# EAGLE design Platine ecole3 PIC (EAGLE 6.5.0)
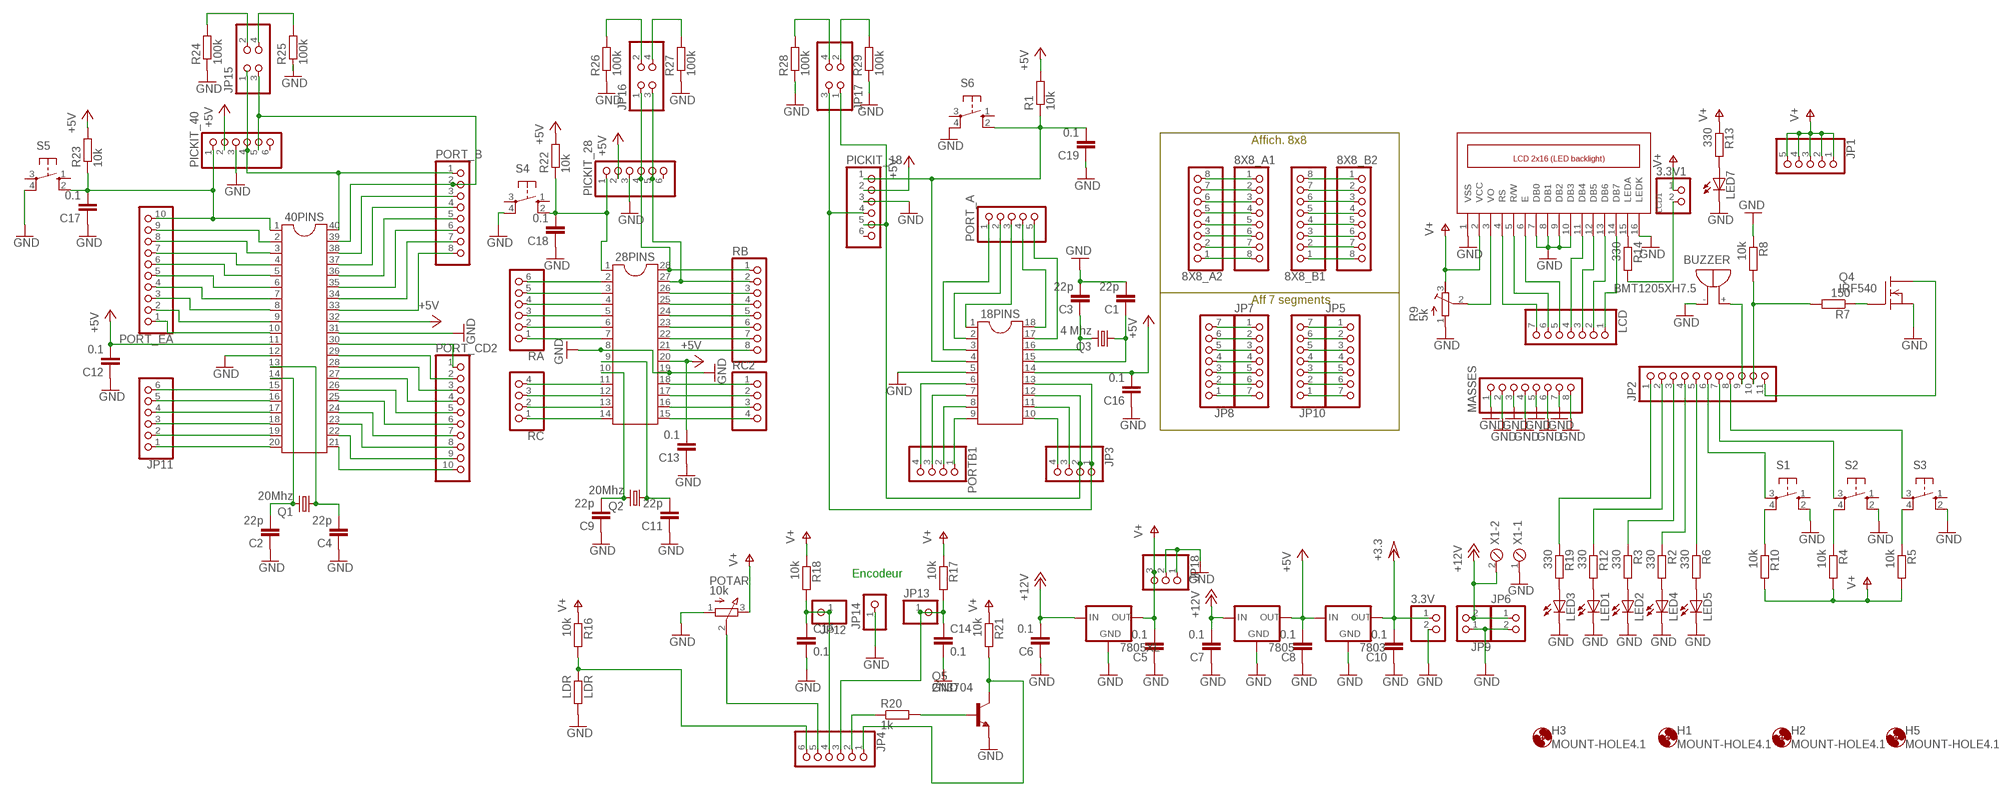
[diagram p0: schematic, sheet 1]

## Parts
3.3V  PINHD-1X2  [1X02]
3.3V1  PINHD-1X2  [1X02]
8X8_A1  PINHD-1X8/LONG  [1X08]
8X8_A2  PINHD-1X8/LONG  [1X08]
8X8_B1  PINHD-1X8/LONG  [1X08]
8X8_B2  PINHD-1X8/LONG  [1X08]
18PINS  DIL18  [DIL18]
28PINS  DIL28-3  [DIL28-3]
40PINS  DIL40  [DIL40]
7803  78LXX  [78LXX]
7805  78LXX  [78LXX]
7805XL  78XXL  [78XXL]
BUZZER  BMT1205XH7.5  [BMT1205XH7.5]
C1  22p  C-EU050-025X075  [C050-025X075]
C2  22p  C-EU050-025X075  [C050-025X075]
C3  22p  C-EU050-025X075  [C050-025X075]
C4  22p  C-EU050-025X075  [C050-025X075]
C5  0.1  C-EU050-025X075  [C050-025X075]
C6  0.1  C-EU050-025X075  [C050-025X075]
C7  0.1  C-EU050-025X075  [C050-025X075]
C8  0.1  C-EU050-025X075  [C050-025X075]
C9  22p  C-EU050-025X075  [C050-025X075]
C10  0.1  C-EU050-025X075  [C050-025X075]
C11  22p  C-EU050-025X075  [C050-025X075]
C12  0.1  C-EU050-025X075  [C050-025X075]
C13  0.1  C-EU050-025X075  [C050-025X075]
C14  0.1  C-EU075-032X103  [C075-032X103]
C15  0.1  C-EU075-032X103  [C075-032X103]
C16  0.1  C-EU050-025X075  [C050-025X075]
C17  0.1  C-EU050-025X075  [C050-025X075]
C18  0.1  C-EU050-025X075  [C050-025X075]
C19  0.1  C-EU050-025X075  [C050-025X075]
H1  MOUNT-HOLE4.1  [4,1]
H2  MOUNT-HOLE4.1  [4,1]
H3  MOUNT-HOLE4.1  [4,1]
H5  MOUNT-HOLE4.1  [4,1]
JP1  PINHD-1X5  [1X05]
JP2  PINHD-1X11  [1X11]
JP3  PINHD-1X4  [1X04]
JP4  PINHD-1X6  [1X06]
JP5  PINHD-1X7  [1X07]
JP6  PINHD-1X2  [1X02]
JP7  PINHD-1X7  [1X07]
JP8  PINHD-1X7  [1X07]
JP9  PINHD-1X2  [1X02]
JP10  PINHD-1X7  [1X07]
JP11  PINHD-1X6  [1X06]
JP12  PINHD-1X1  [1X01]
JP13  PINHD-1X1  [1X01]
JP14  PINHD-1X1  [1X01]
JP15  PINHD-2X2  [2X02]
JP16  PINHD-2X2  [2X02]
JP17  PINHD-2X2  [2X02]
JP18  PINHD-1X3  [1X03]
LCD  PINHD-1X7/LONG  [1X07]
LCD1  LCD_2X16_SIL  [HY-1602F]
LDR  LDR  R-EU_0207/7  [0207/7]
LED1  LED5MM  [LED5MM]
LED2  LED5MM  [LED5MM]
LED3  LED5MM  [LED5MM]
LED4  LED5MM  [LED5MM]
LED5  LED5MM  [LED5MM]
LED7  LED3MM  [LED3MM]
MASSES  PINHD-1X8/LONG  [1X08]
PICKIT_18  PINHD-1X6  [1X06]
PICKIT_28  PINHD-1X6  [1X06]
PICKIT_40  PINHD-1X6  [1X06]
PORT_A  PINHD-1X5  [1X05]
PORT_B  PINHD-1X8  [1X08]
PORT_CD2  PINHD-1X10  [1X10]
PORT_EA  PINHD-1X10  [1X10]
PORTB1  PINHD-1X4  [1X04]
POTAR  10k  EVUF2A  [EVUF]
Q1  20Mhz  CRYSTALHC49S  [HC49/S]
Q2  20Mhz  CRYSTALHC49S  [HC49/S]
Q3  4 Mhz  CRYSTALHC49S  [HC49/S]
Q4  IRF540  [TO220]
Q5  2N3704  [TO92]
R1  10k  R-EU_0207/7  [0207/7]
R2  330  R-EU_0207/7  [0207/7]
R3  330  R-EU_0207/7  [0207/7]
R4  10k  R-EU_0207/7  [0207/7]
R5  10k  R-EU_0207/7  [0207/7]
R6  330  R-EU_0207/7  [0207/7]
R7  150  R-EU_0207/7  [0207/7]
R8  10k  R-EU_0207/7  [0207/7]
R9  5k  R-TRIMM3339P  [RTRIM3339P]
R10  10k  R-EU_0207/7  [0207/7]
R12  330  R-EU_0207/7  [0207/7]
R13  330  R-EU_0207/7  [0207/7]
R14  330  R-EU_0207/7  [0207/7]
R16  10k  R-EU_0207/7  [0207/7]
R17  10k  R-EU_0207/7  [0207/7]
R18  10k  R-EU_0207/7  [0207/7]
R19  330  R-EU_0207/7  [0207/7]
R20  1k  R-EU_0207/7  [0207/7]
R21  10k  R-EU_0207/7  [0207/7]
R22  10k  R-EU_0207/7  [0207/7]
R23  10k  R-EU_0207/7  [0207/7]
R24  100k  R-EU_0207/7  [0207/7]
R25  100k  R-EU_0207/7  [0207/7]
R26  100k  R-EU_0207/7  [0207/7]
R27  100k  R-EU_0207/7  [0207/7]
R28  100k  R-EU_0207/7  [0207/7]
R29  100k  R-EU_0207/7  [0207/7]
RA  PINHD-1X6  [1X06]
RB  PINHD-1X8  [1X08]
RC  PINHD-1X4  [1X04]
RC2  PINHD-1X4  [1X04]
S1  10-XX  [B3F-10XX]
S2  10-XX  [B3F-10XX]
S3  10-XX  [B3F-10XX]
S4  10-XX  [B3F-10XX]
S5  10-XX  [B3F-10XX]
S6  10-XX  [B3F-10XX]
X1  MPT2  [2POL254]

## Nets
8X8_A1: 8X8_A1.1 8X8_A2.8
+5V: 18PINS.14 28PINS.20 40PINS.11 40PINS.32 7803.IN 7805.OUT C8.2 C12.2 C13.2 C16.2 PICKIT_18.2 PICKIT_28.2 PICKIT_40.2 R1.2 R22.2 R23.2
+12V: 7805.IN 7805XL.IN C6.2 C7.2 JP6.1 JP9.2 X1.2
GND: 3.3V.2 18PINS.5 28PINS.8 28PINS.19 40PINS.12 40PINS.31 7803.GND 7805.GND 7805XL.GND BUZZER.- C1.2 C2.1 C3.2 C4.1 C5.1 C6.1 C7.1 C8.1 C9.1 C10.1 C11.1 C12.1 C13.1 C14.2 C15.2 C16.1 C17.1 C18.1 C19.1 JP6.2 JP9.1 JP14.1 JP18.1 JP18.2 LCD1.1(VSS) LCD1.7(DB0) LCD1.8(DB1) LCD1.9(DB2) LCD1.10(DB3) LCD1.16(LEDK) LDR.2 LED1.K(C) LED2.K(C) LED3.K(C) LED4.K(C) LED5.K(C) LED7.K(C) MASSES.1 MASSES.2 MASSES.3 MASSES.4 MASSES.5 MASSES.6 MASSES.7 MASSES.8 PICKIT_18.3 PICKIT_28.3 PICKIT_40.3 POTAR.1(A) Q4.3(S) Q5.3(E) R8.1 R9.1(A) R24.1 R25.1 R26.1 R27.1 R28.1 R29.1 S1.2(S1) S2.2(S1) S3.2(S1) S4.4(P1) S5.4(P1) S6.4(P1) X1.1
LED_POUSS: JP2.2 R12.1
N$1: 18PINS.16 C3.1 Q3.2
N$2: 18PINS.11 JP3.3
N$3: 18PINS.15 C1.1 Q3.1
N$4: 18PINS.10 JP3.4
N$5: 18PINS.13 JP3.1 JP17.3 PICKIT_18.4
N$7: 18PINS.9 PORTB1.1
N$9: 18PINS.7 PORTB1.3
N$10: 18PINS.6 PORTB1.4
N$11: 18PINS.17 PORT_A.5
N$12: 18PINS.18 PORT_A.4
N$13: 18PINS.1 PORT_A.3
N$14: 18PINS.2 PORT_A.2
N$15: 18PINS.3 PORT_A.1
N$16: 40PINS.40 JP15.1 PICKIT_40.4 PORT_B.1
N$17: 18PINS.4 C19.2 PICKIT_18.1 R1.1 S6.2(S1)
N$18: 40PINS.39 JP15.3 PICKIT_40.5 PORT_B.2
N$19: 40PINS.1 C17.2 PICKIT_40.1 PORT_EA.10 R23.1 S5.2(S1)
N$20: LED1.A R12.2
N$21: R4.1 S2.4(P1)
N$22: JP2.11 Q4.2(D)
N$23: R5.1 S3.4(P1)
N$24: LED2.A R3.2
N$25: LED4.A R2.2
N$26: LED5.A R6.2
N$27: R10.1 S1.4(P1)
N$29: JP2.7 S2.3(P)
N$30: JP2.8 S3.3(P)
N$31: JP2.10 R7.2 R8.2
N$32: Q4.1(G) R7.1
N$33: 40PINS.2 PORT_EA.9
N$34: 40PINS.3 PORT_EA.8
N$35: 40PINS.4 PORT_EA.7
N$36: 40PINS.5 PORT_EA.6
N$37: 40PINS.6 PORT_EA.5
N$38: 40PINS.7 PORT_EA.4
N$39: 40PINS.8 PORT_EA.3
N$40: 40PINS.9 PORT_EA.2
N$41: 40PINS.10 PORT_EA.1
N$42: BUZZER.+ JP2.9
N$68: 40PINS.38 PORT_B.3
N$69: 40PINS.37 PORT_B.4
N$70: 40PINS.36 PORT_B.5
N$71: 40PINS.35 PORT_B.6
N$72: 40PINS.34 PORT_B.7
N$73: 40PINS.33 PORT_B.8
N$74: 40PINS.15 JP11.6
N$75: 40PINS.16 JP11.5
N$76: 40PINS.17 JP11.4
N$77: 40PINS.19 JP11.2
N$78: 40PINS.20 JP11.1
N$79: 40PINS.30 PORT_CD2.1
N$80: 40PINS.29 PORT_CD2.2
N$81: 40PINS.27 PORT_CD2.4
N$82: 40PINS.28 PORT_CD2.3
N$83: 40PINS.26 PORT_CD2.5
N$84: 40PINS.25 PORT_CD2.6
N$85: 40PINS.24 PORT_CD2.7
N$86: 40PINS.23 PORT_CD2.8
N$87: 40PINS.22 PORT_CD2.9
N$88: 40PINS.21 PORT_CD2.10
N$89: LCD1.3(VO) R9.2(S)
N$90: 40PINS.14 C2.2 Q1.2
N$91: 40PINS.13 C4.2 Q1.1
N$93: 8X8_A1.2 8X8_A2.7
N$94: 8X8_A1.3 8X8_A2.6
N$95: 8X8_A1.4 8X8_A2.5
N$96: 8X8_A1.5 8X8_A2.4
N$97: 8X8_A1.6 8X8_A2.3
N$98: 8X8_A1.7 8X8_A2.2
N$99: 8X8_A1.8 8X8_A2.1
N$100: 8X8_B1.8 8X8_B2.1
N$101: 8X8_B1.7 8X8_B2.2
N$102: 8X8_B1.6 8X8_B2.3
N$103: 8X8_B1.5 8X8_B2.4
N$104: 8X8_B1.4 8X8_B2.5
N$105: 8X8_B1.3 8X8_B2.6
N$106: 8X8_B1.2 8X8_B2.7
N$107: 8X8_B1.1 8X8_B2.8
N$108: LCD1.11(DB4) LCD.4
N$109: LCD1.4(RS) LCD.7
N$110: LCD1.5(R/W) LCD.6
N$111: LCD1.6(E) LCD.5
N$112: LCD1.12(DB5) LCD.3
N$113: LCD1.13(DB6) LCD.2
N$114: LCD1.14(DB7) LCD.1
N$116: JP2.5 R6.1
N$117: JP2.6 S1.3(P)
N$118: JP2.4 R2.1
N$119: JP2.3 R3.1
N$143: LED7.A R13.2
N$144: LCD1.15(LEDA) R14.1
N$145: 3.3V1.2 R14.2
N$148: JP7.1 JP8.7
N$149: JP7.2 JP8.6
N$150: JP7.3 JP8.5
N$151: JP7.4 JP8.4
N$152: JP7.5 JP8.3
N$153: JP5.1 JP10.7
N$154: JP5.2 JP10.6
N$155: JP5.3 JP10.5
N$156: JP5.4 JP10.4
N$157: JP5.5 JP10.3
N$158: JP7.6 JP8.2
N$159: JP7.7 JP8.1
N$160: JP5.6 JP10.2
N$161: JP5.7 JP10.1
N$166: 28PINS.10 C9.2 Q2.2
N$167: 28PINS.9 C11.2 Q2.1
N$168: 28PINS.2 RA.6
N$170: 28PINS.3 RA.5
N$171: 28PINS.28 JP16.1 PICKIT_28.4 RB.1
N$172: 28PINS.27 JP16.3 PICKIT_28.5 RB.2
N$173: 28PINS.4 RA.4
N$174: 28PINS.5 RA.3
N$175: 28PINS.6 RA.2
N$176: 28PINS.7 RA.1
N$177: 28PINS.11 RC.4
N$178: 28PINS.12 RC.3
N$179: 28PINS.13 RC.2
N$180: 28PINS.14 RC.1
N$181: 28PINS.18 RC2.1
N$182: 28PINS.17 RC2.2
N$183: 28PINS.16 RC2.3
N$184: 28PINS.15 RC2.4
N$185: 28PINS.21 RB.8
N$186: 28PINS.22 RB.7
N$187: 28PINS.23 RB.6
N$188: 28PINS.24 RB.5
N$189: 28PINS.25 RB.4
N$190: 28PINS.26 RB.3
N$196: JP4.5 POTAR.2(S)
N$197: C14.1 JP4.3 JP13.1 R17.2
N$198: C15.1 JP4.4 JP12.1 R18.2
N$199: JP4.6 LDR.1 R16.2
N$206: LED3.A R19.2
N$207: JP2.1 R19.1
N$208: JP4.1 Q5.2(C) R21.2
N$209: Q5.1(B) R20.2
N$210: JP4.2 R20.1
N$211: 40PINS.18 JP11.3
N$213: 28PINS.1 C18.2 PICKIT_28.1 R22.1 S4.2(S1)
N$216: JP15.2 R24.2
N$217: JP15.4 R25.2
N$222: JP16.2 R26.2
N$223: JP16.4 R27.2
N$224: JP17.4 R28.2
N$225: JP17.2 R29.2
PORT_B84: 18PINS.8 PORTB1.2
PORTB2: 18PINS.12 JP3.2 JP17.1 PICKIT_18.5
V+: 3.3V1.1 7805XL.OUT C5.2 JP1.1 JP1.2 JP1.3 JP1.4 JP1.5 JP18.3 LCD1.2(VCC) POTAR.3(E) R4.2 R5.2 R9.3(E) R10.2 R13.1 R16.1 R17.1 R18.1 R21.1
VCC/2: 3.3V.1 7803.OUT C10.2 ; supply symbol labelled +3.3
Unconnected: PICKIT_18.6 PICKIT_28.6 PICKIT_40.6 S1.1(S) S2.1(S) S3.1(S) S4.1(S) S4.3(P) S5.1(S) S5.3(P) S6.1(S) S6.3(P)

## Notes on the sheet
- Affich. 8x8
- Aff 7 segments
- Encodeur

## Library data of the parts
3.3V 3.3V1 JP6 JP9 = pinhead:PINHD-1X2: PIN HEADER
8X8_A1 8X8_A2 8X8_B1 8X8_B2 MASSES = pinhead_v2:PINHD-1X8: PIN HEADER
18PINS = ic-package:DIL18: Dual In Line / Socket
28PINS = ic-package:DIL28: Dual In Line
40PINS = ic-package:DIL40: Dual In Line
7803 7805 = v-reg:78LXX: VOLTAGE REGULATOR
7805XL = v-reg:78XXL: VOLTAGE REGULATOR
BUZZER = buzzer:BMT1205XH7.5: MAGNETIC TRANSDUCER; OC_FARNELL: unknown; OC_NEWARK: unknown
C1-C19 = rcl:C-EU: CAPACITOR, European symbol
H1-H3 H5 = holes:MOUNT-HOLE: MOUNTING HOLE with drill center marker
JP1 PORT_A = pinhead:PINHD-1X5: PIN HEADER
JP2 = pinhead:PINHD-1X11: PIN HEADER
JP3 PORTB1 RC RC2 = pinhead:PINHD-1X4: PIN HEADER
JP4 JP11 PICKIT_18 PICKIT_28 PICKIT_40 RA = pinhead:PINHD-1X6: PIN HEADER
JP5 JP7 JP8 JP10 = pinhead:PINHD-1X7: PIN HEADER
JP12-JP14 = pinhead:PINHD-1X1: PIN HEADER
JP15-JP17 = pinhead:PINHD-2X2: PIN HEADER
JP18 = pinhead:PINHD-1X3: PIN HEADER
LCD = pinhead_v2:PINHD-1X7: PIN HEADER
LCD1 = lcd_2x16_led_backlight:LCD_2X16_SIL
LDR R1-R8 R10 R12-R14 R16-R29 = rcl:R-EU_: RESISTOR, European symbol
LED1-LED5 LED7 = led:LED: LED
PORT_B RB = pinhead:PINHD-1X8: PIN HEADER
PORT_CD2 PORT_EA = pinhead:PINHD-1X10: PIN HEADER
POTAR = pot:EVU: 9 mm Square Rotary Potentiometers Source: Panasonic
Q1-Q3 = crystal:CRYSTAL: CRYSTAL
Q4 = transistor-fet:IRF540: N-Channel Enhancement MOSFET (HEXFET); 100V; 28A; 0,077Ohm
Q5 = transistor-npn:2N3704: NPN Transistor
R9 = rcl:R-TRIMM: Trimm resistor
S1-S6 = switch-omron:10-XX: OMRON SWITCH; MPN: B3F-1000; OC_FARNELL: 176432; OC_NEWARK: 36M3542
X1 = con-phoenix-254:MPT2: PHOENIX CONNECTOR; OC_FARNELL: unknown; OC_NEWARK: unknown

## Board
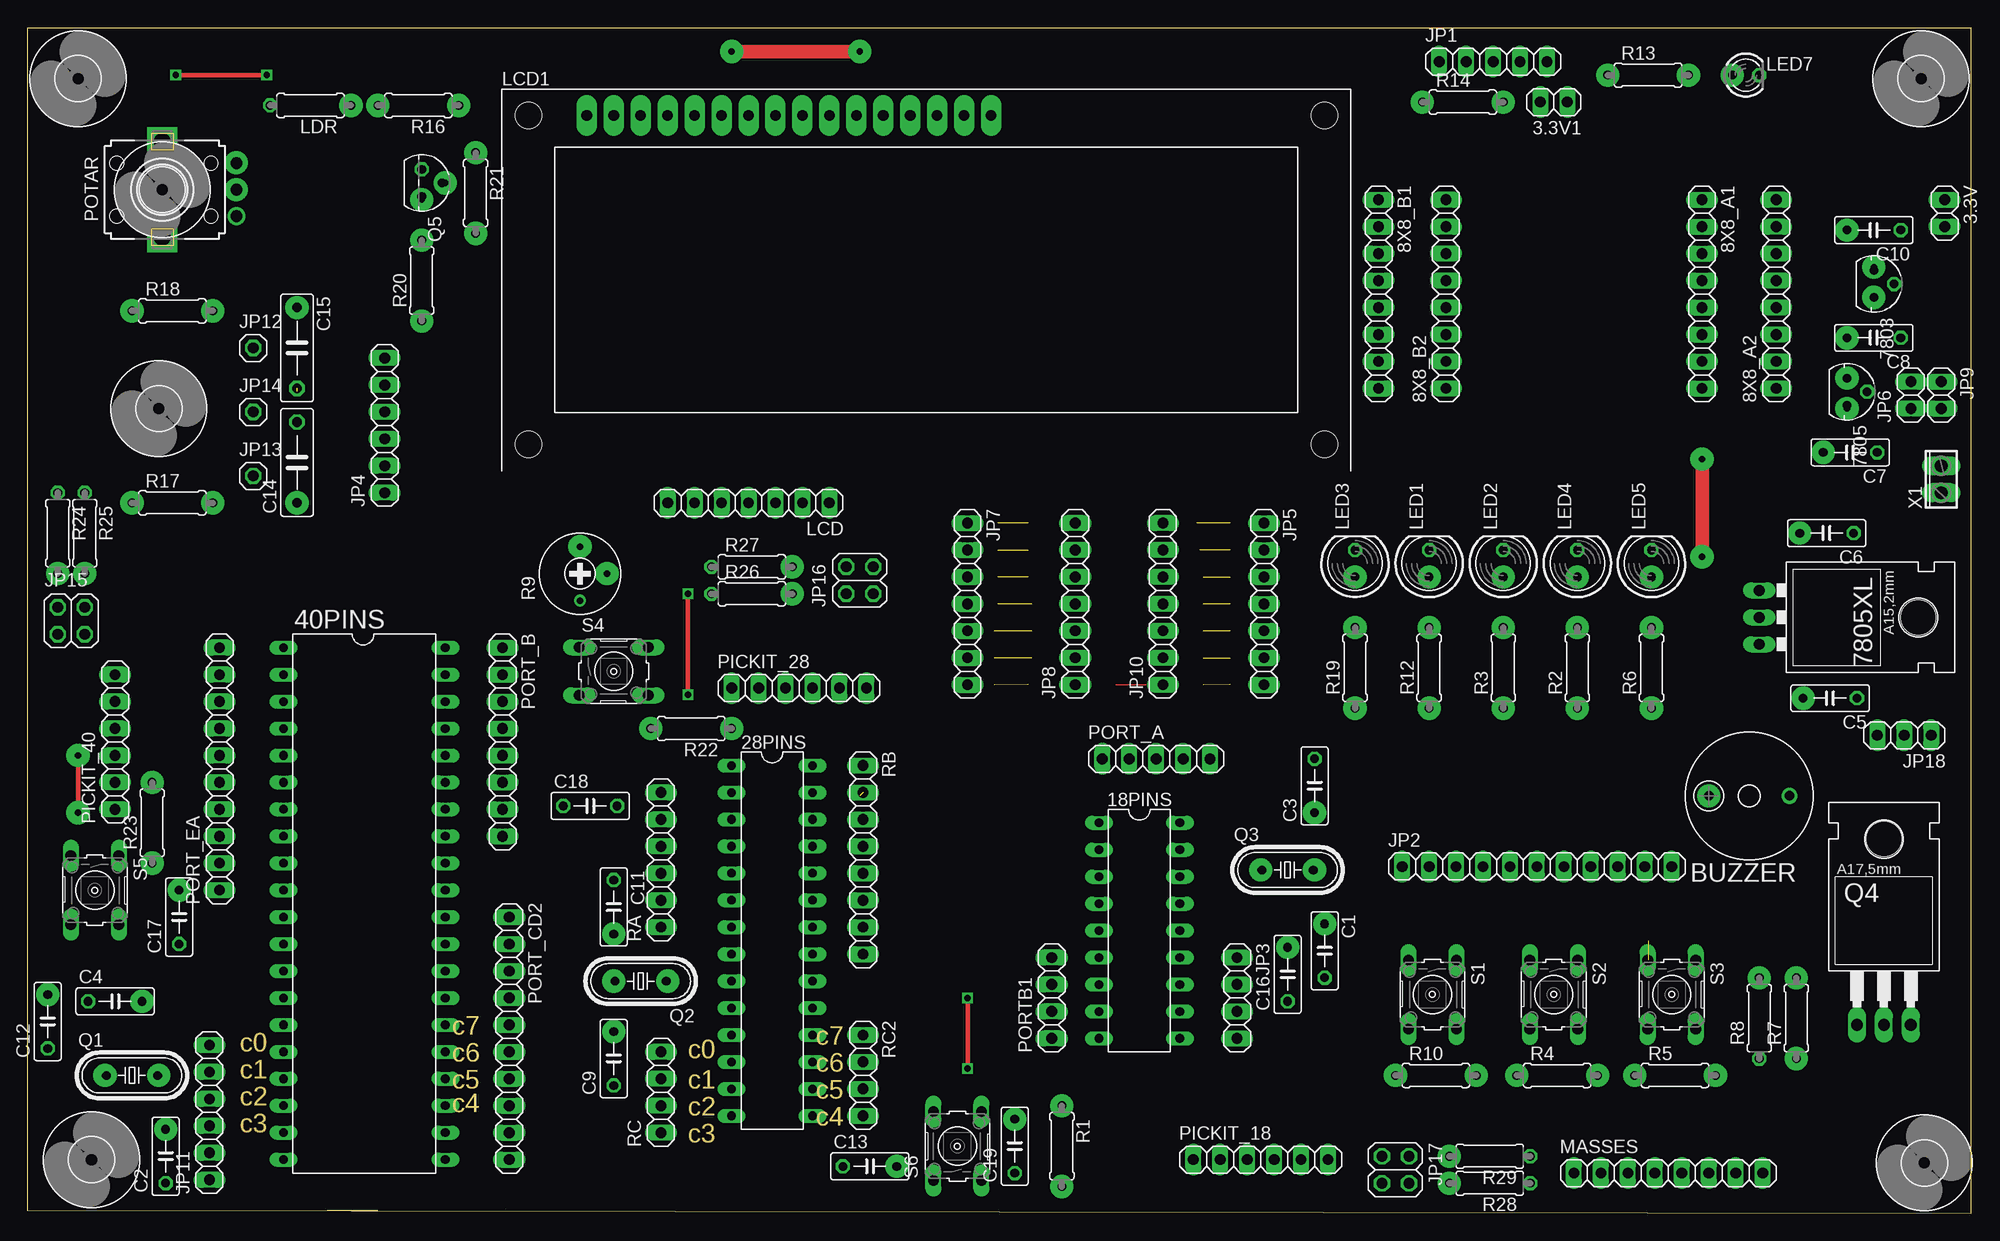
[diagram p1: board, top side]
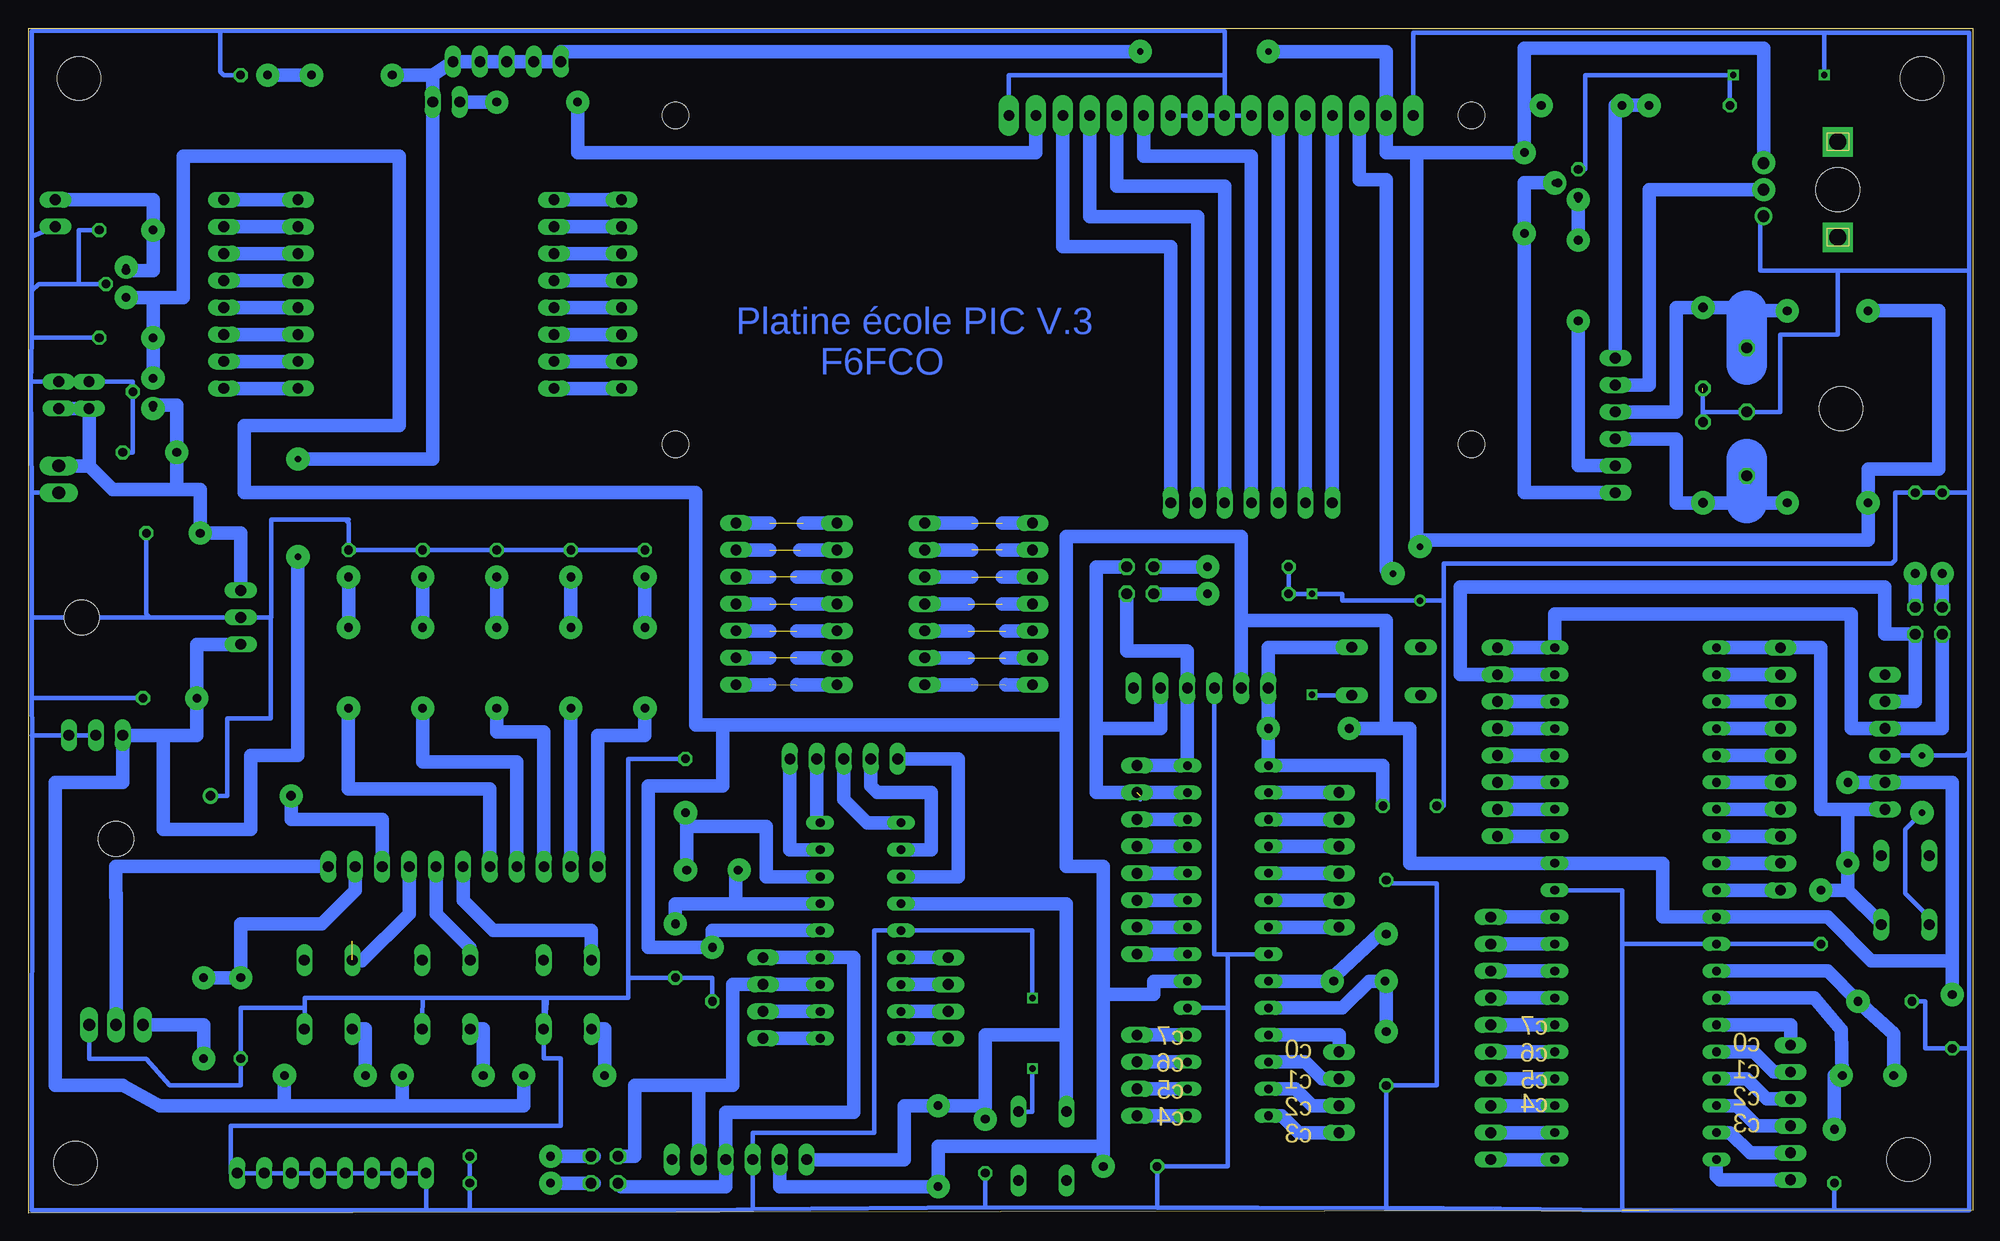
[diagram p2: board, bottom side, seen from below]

Size 183.18 x 111.75 mm. Coordinates in mm from the lower left corner, seen from the top.
Outline: 0,0.32 183.18,0 183.18,111.75 0,111.75 0,0.32
Copper layers (1*16): Top 0.035mm / dielectric 1.5mm / Bottom 0.035mm
Design rules "default": minimum track width 10mil, minimum drill 24mil, track to track 8mil, track to pad 8mil, pad to pad 8mil, via to via 8mil, smd to smd 8mil, copper to edge 40mil, drill to drill 8mil, minimum pad ring 10mil, minimum via ring 8mil, stop-mask expansion 4mil, vias tented up to drill 0mil, thermal gap 10mil

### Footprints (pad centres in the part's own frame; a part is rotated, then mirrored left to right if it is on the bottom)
1X02 = drill 1.016 long: 1 -1.27,0; 2 1.27,0
1X08 = drill 1.016 long: 1 -8.89,0; 2 -6.35,0; 3 -3.81,0; 4 -1.27,0; 5 1.27,0; 6 3.81,0; 7 6.35,0; 8 8.89,0
DIL18 = drill 0.813 long: 1 -10.16,-3.81; 2 -7.62,-3.81; 3 -5.08,-3.81; 4 -2.54,-3.81; 5 0,-3.81; 6 2.54,-3.81; 7 5.08,-3.81; 8 7.62,-3.81; 9 10.16,-3.81; 10 10.16,3.81; 11 7.62,3.81; 12 5.08,3.81; 13 2.54,3.81; 14 0,3.81; 15 -2.54,3.81; 16 -5.08,3.81; 17 -7.62,3.81; 18 -10.16,3.81
DIL28-3 = drill 0.813 long: 1 -16.51,-3.81; 2 -13.97,-3.81; 3 -11.43,-3.81; 4 -8.89,-3.81; 5 -6.35,-3.81; 6 -3.81,-3.81; 7 -1.27,-3.81; 8 1.27,-3.81; 9 3.81,-3.81; 10 6.35,-3.81; 11 8.89,-3.81; 12 11.43,-3.81; 13 13.97,-3.81; 14 16.51,-3.81; 15 16.51,3.81; 16 13.97,3.81; 17 11.43,3.81; 18 8.89,3.81; 19 6.35,3.81; 20 3.81,3.81; 21 1.27,3.81; 22 -1.27,3.81; 23 -3.81,3.81; 24 -6.35,3.81; 25 -8.89,3.81; 26 -11.43,3.81; 27 -13.97,3.81; 28 -16.51,3.81
DIL40 = drill 0.813 long: 1 -24.13,-7.62; 2 -21.59,-7.62; 3 -19.05,-7.62; 4 -16.51,-7.62; 5 -13.97,-7.62; 6 -11.43,-7.62; 7 -8.89,-7.62; 8 -6.35,-7.62; 9 -3.81,-7.62; 10 -1.27,-7.62; 11 1.27,-7.62; 12 3.81,-7.62; 13 6.35,-7.62; 14 8.89,-7.62; 15 11.43,-7.62; 16 13.97,-7.62; 17 16.51,-7.62; 18 19.05,-7.62; 19 21.59,-7.62; 20 24.13,-7.62; 21 24.13,7.62; 22 21.59,7.62; 23 19.05,7.62; 24 16.51,7.62; 25 13.97,7.62; 26 11.43,7.62; 27 8.89,7.62; 28 6.35,7.62; 29 3.81,7.62; 30 1.27,7.62; 31 -1.27,7.62; 32 -3.81,7.62; 33 -6.35,7.62; 34 -8.89,7.62; 35 -11.43,7.62; 36 -13.97,7.62; 37 -16.51,7.62; 38 -19.05,7.62; 39 -21.59,7.62; 40 -24.13,7.62
78LXX = drill 0.813 octagon: GND 0,1.905; IN 1.27,0; OUT -1.27,0
78XXL = drill 1.016 long: GND 0,-3.81; IN -2.54,-3.81; OUT 2.54,-3.81 | hole 3.302: 0,11.176
BMT1205XH7.5 = drill 0.9 pad 1.5: + 3.8,0; - -3.8,0
C050-025X075 = drill 0.813 octagon: 1 -2.54,0; 2 2.54,0
C075-032X103 = drill 0.914 octagon: 1 -3.81,0; 2 3.81,0
4,1 = hole 4.1: 0,0
1X05 = drill 1.016 long: 1 -5.08,0; 2 -2.54,0; 3 0,0; 4 2.54,0; 5 5.08,0
1X11 = drill 1.016 long: 1 -12.7,0; 2 -10.16,0; 3 -7.62,0; 4 -5.08,0; 5 -2.54,0; 6 0,0; 7 2.54,0; 8 5.08,0; 9 7.62,0; 10 10.16,0; 11 12.7,0
1X04 = drill 1.016 long: 1 -3.81,0; 2 -1.27,0; 3 1.27,0; 4 3.81,0
1X06 = drill 1.016 long: 1 -6.35,0; 2 -3.81,0; 3 -1.27,0; 4 1.27,0; 5 3.81,0; 6 6.35,0
1X07 = drill 1.016 long: 1 -7.62,0; 2 -5.08,0; 3 -2.54,0; 4 0,0; 5 2.54,0; 6 5.08,0; 7 7.62,0
1X01 = drill 1.016 octagon: 1 0,0
2X02 = drill 1.016 octagon: 1 -1.27,-1.27; 2 -1.27,1.27; 3 1.27,-1.27; 4 1.27,1.27
1X03 = drill 1.016 long: 1 -2.54,0; 2 0,0; 3 2.54,0
HY-1602F = drill 1 pad 1.93 long: 1 2.54,0; 2 5.08,0; 3 7.62,0; 4 10.16,0; 5 12.7,0; 6 15.24,0; 7 17.78,0; 8 20.32,0; 9 22.86,0; 10 25.4,0; 11 27.94,0; 12 30.48,0; 13 33.02,0; 14 35.56,0; 15 38.1,0; 16 40.64,0 | hole 2.5: -2.96,0; 72.04,0; -2.96,-31; 72.04,-31
0207/7 = drill 0.813 octagon: 1 -3.81,0; 2 3.81,0
LED5MM = drill 0.813 octagon: A -1.27,0; K 1.27,0
LED3MM = drill 0.813 octagon: A -1.27,0; K 1.27,0
1X10 = drill 1.016 long: 1 -11.43,0; 2 -8.89,0; 3 -6.35,0; 4 -3.81,0; 5 -1.27,0; 6 1.27,0; 7 3.81,0; 8 6.35,0; 9 8.89,0; 10 11.43,0
EVUF = drill 1.1 pad 1.676: 1 -2.5,-7; 2 0,-7; 3 2.5,-7 | drill 1.6 pad 2.8 square: M1 4.5,0; M2 -4.5,0
HC49/S = drill 0.813: 1 -2.413,0; 2 2.413,0
TO220 = drill 1.118 long: 1 -2.54,-6.35; 2 0,-6.35; 3 2.54,-6.35 | hole 3.302: 0,11.176
TO92 = drill 0.813 octagon: 1 1.27,0; 2 0,1.905; 3 -1.27,0
RTRIM3339P = drill 0.61: 1 -2.54,0; 2 0,-2.54; 3 2.54,0
B3F-10XX = drill 1.016 long: 1 -3.251,2.261; 2 3.251,2.261; 3 -3.251,-2.261; 4 3.251,-2.261
2POL254 = drill 1.2 long: 1 -1.27,0; 2 1.27,0

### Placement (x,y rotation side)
3.3V  180.66,94.31 270 top
3.3V1  143.83,104.78 180 top
8X8_A1  157.8,86.68 270 top
8X8_A2  164.78,86.68 90 top
8X8_B1  127.32,86.68 270 top
8X8_B2  133.67,86.68 90 top
18PINS  104.78,26.67 270 top
28PINS  70.17,25.72 270 top
40PINS  31.75,29.21 270 top
7803  173.99,87.63 270 top
7805  171.45,77.47 270 top
7805XL  167.01,56.2 270 top
BUZZER  162.24,39.37 180 top
C1  122.24,24.77 270 top
C2  13.02,5.4 90 top
C3  121.29,40.32 90 top
C4  8.25,20 0 top
C5  169.86,48.58 180 top
C6  169.55,64.14 180 top
C7  171.77,71.76 180 top
C8  173.99,82.55 180 top
C9  55.25,14.61 90 top
C10  173.99,92.71 180 top
C11  55.25,28.89 270 top
C12  1.9,18.1 90 top
C13  79.38,4.45 0 top
C14  25.4,70.8 90 top
C15  25.4,81.6 270 top
C16  118.75,22.54 90 top
C17  14.29,27.94 90 top
C18  53.02,38.42 0 top
C19  93.03,6.35 90 top
H1  178.44,107 0 top
H2  178.75,4.76 0 top
H3  6.03,5.08 0 top
H4  MOUNT-HOLE4.1  [4,1]  4.76,107 0 top
H5  12.7,96.52 0 top
H6  MOUNT-HOLE4.1  [4,1]  12.38,75.88 0 top
JP1  138.12,108.59 0 top
JP2  142.24,32.7 0 top
JP3  113.98,20.32 270 top
JP4  33.66,74.3 90 top
JP5  116.52,57.47 270 top
JP6  177.48,77.15 90 top
JP7  88.58,57.47 270 top
JP8  98.74,57.47 90 top
JP9  180.34,77.15 270 top
JP10  107,57.47 90 top
JP11  17.15,9.53 90 top
JP12  21.27,81.6 0 top
JP13  21.27,69.53 0 top
JP14  21.27,75.57 0 top
JP15  4.13,55.88 0 top
JP16  78.42,59.69 90 top
JP17  128.91,4.13 270 top
JP18  176.85,45.09 180 top
LCD  67.95,66.99 180 top
LCD1  50.17,103.5 0 top
LDR  26.67,104.46 180 top
LED1  132.08,61.28 90 top
LED2  139.07,61.28 90 top
LED3  125.1,61.28 90 top
LED4  146.05,61.28 90 top
LED5  153.04,61.28 90 top
LED7  161.93,107.32 0 top
MASSES  154.62,3.81 0 top
PICKIT_18  116.21,5.08 0 top
PICKIT_28  72.71,49.53 0 top
PICKIT_40  8.26,44.45 90 top
PORT_A  106.36,42.86 0 top
PORT_B  44.77,44.45 270 top
PORT_CD2  45.4,16.51 270 top
PORT_EA  18.1,41.91 90 top
PORTB1  96.52,20.32 90 top
POTAR  12.7,96.52 90 top
Q1  9.84,13.02 0 top
Q2  57.79,21.91 180 top
Q3  118.75,32.39 0 top
Q4  174.94,24.13 0 top
Q5  37.15,97.16 270 top
R1  97.48,6.35 270 top
R2  146.05,51.44 90 top
R3  139.07,51.44 90 top
R4  144.15,13.01 0 top
R5  155.26,13.01 0 top
R6  153.04,51.44 90 top
R7  166.69,18.41 90 top
R8  163.2,18.41 90 top
R9  52.07,60.32 90 top
R10  132.72,13.02 0 top
R12  132.08,51.44 90 top
R13  152.72,107.32 0 top
R14  135.26,104.78 0 top
R16  36.83,104.46 180 top
R17  13.65,66.99 0 top
R18  13.65,85.09 0 top
R19  125.1,51.44 90 top
R20  37.15,87.95 90 top
R21  42.23,96.21 270 top
R22  62.55,45.72 180 top
R23  11.75,36.83 90 top
R24  2.86,64.14 270 top
R25  5.4,64.14 270 top
R26  68.26,58.42 0 top
R27  68.26,60.96 0 top
R28  137.8,2.86 180 top
R29  137.8,5.4 180 top
RA  59.69,33.34 90 top
RB  78.74,33.34 270 top
RC  59.69,11.43 90 top
RC2  78.74,13.02 270 top
S1  132.4,20.64 270 top
S2  143.83,20.64 270 top
S3  154.94,20.64 270 top
S4  55.25,51.12 0 top
S5  6.35,30.48 270 top
S6  87.63,6.35 90 top
X1  180.34,69.22 90 top

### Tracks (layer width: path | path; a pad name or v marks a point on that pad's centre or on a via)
8X8_A1
  Bottom 1.27: 8X8_A1.1 8X8_A2.8
+5V  (via drill 0.6 pad 2.18)
  Bottom 1.27: 81.92,20.64 | 81.92,20.64 81.92,5.08 C13.2 | 112.4,3.49 PICKIT_18.2 112.4,2.54 101.6,2.54 R1.2 | 18PINS.14 118.75,26.67 C16.2 | C16.2 124.78,25.08 124.78,40.32 117.79,40.32 117.79,46.04 117.8,46.04 | 7805.OUT C8.2 171.45,86.36 172.09,86.36 | 7805.OUT | 7803.IN 172.09,86.36 | 172.09,86.36 168.6,86.36 168.6,99.7 148.28,99.7 148.28,74.3 162.88,74.3 162.88,67.94 120.33,67.94 120.33,66.67 120.33,46.04 117.8,46.04 | 55.25,45.72 53.02,45.72 53.02,33.02 40PINS.32 29.21,33.02 29.21,27.94 28.58,27.94 28.57,27.94 40PINS.11 13.65,27.94 9.52,23.81 1.9,23.81 | 55.25,45.72 R22.2 | R22.2 | 28PINS.20 77.15,21.91 77.15,20.64 81.92,20.64 | PICKIT_40.2 7.94,40.64 1.9,40.64 | 1.9,40.64 R23.2 | 1.9,40.64 1.9,38.1 1.9,29.85 | 1.9,29.85 1.9,27.94 | R22.2 | R22.2 | C12.2 1.9,21.91 1.9,23.81 | 1.9,23.81 1.9,29.85 | C13.2 | C13.2 81.92,6.35 84.46,6.35 92.39,6.35 95.25,6.35 97.48,6.35 R1.2 | C16.2 | 68.9,55.88 55.25,55.88 55.25,45.72 | 68.9,55.88 | 68.9,55.88 PICKIT_28.2 | 85.41,46.67 85.41,46.36 85.41,32.7 81.92,32.7 81.92,20.64 | 85.41,46.67 85.41,63.82 68.9,63.82 68.9,55.88 | R1.2 | 81.92,20.64 | 117.8,46.04 85.73,46.04 85.41,46.67 | C13.2 | C13.2
  other vias: 81.92,4.45
+12V
  Bottom 1.27: 7805XL.IN 163.2,64.14 163.83,64.14 C6.2 167.01,68.26 169.23,68.26 C7.2 | 7805.IN 169.23,76.2 C7.2 | JP9.2 JP6.1 177.48,70.49 | 177.48,70.49 X1.2 | 177.48,70.49 175.26,68.26 169.23,68.26 C7.2
GND  (via drill 0.6, 0.6 pad 2.18)  (3 unrouted)
  Top 0.406: v22.54,107.32 v13.97,107.32 | v4.76,37.78 v4.76,43.18 | v62.23,48.9 v62.23,58.42 | v88.58,13.65 v88.58,20.32
  Bottom 0.406: 33.02,25.4 40PINS.12 23.5,25.4 | 33.02,25.4 33.02,0.32 | 165.42,111.49 70.49,111.44 70.49,107.32 | 165.42,111.49 182.88,111.44 182.88,92.07 | 182.88,92.07 182.88,86.99 | 182.88,86.99 182.88,82.55 | 182.88,82.55 182.97,78.11 | 182.97,78.11 182.88,67.94 | 182.88,67.94 182.88,56.2 | 182.88,56.2 182.88,48.58 | 182.88,48.58 182.86,45.08 | 182.86,45.08 182.88,0.32 145.73,0.32 | 145.73,0.32 129.54,0.32 | 129.54,0.32 118.11,0.32 114.93,0.39 | 114.93,0.39 93.03,0.6 | 93.03,0.6 76.84,0.54 | 76.84,0.54 70.17,0.53 67.31,0.52 49.85,0.48 | 49.85,0.48 45.09,0.47 45.4,0.47 45.09,0.47 | 45.09,0.47 44.45,0.45 33.02,0.32 | MASSES.5 MASSES.4 MASSES.3 MASSES.2 MASSES.1 145.73,0.32 | MASSES.5 MASSES.6 MASSES.7 MASSES.8 | LCD1.1 52.71,106.36 52.71,111.31 13.97,111.31 | LCD1.8 LCD1.9 LCD1.10 | LCD1.7 LCD1.8 | LCD1.8 70.49,107.32 | X1.1 182.88,67.94 | C6.1 172.09,56.51 171.77,56.2 | 171.77,56.2 182.88,56.2 | 171.77,56.2 7805XL.GND 160.34,56.2 | C5.1 181.93,48.58 182.88,48.58 | C10.1 178.44,92.71 178.44,87.63 | 178.44,87.63 182.25,87.63 182.88,86.99 | 7803.GND 178.44,87.63 | C8.1 182.88,82.55 | 3.3V.2 182.88,92.07 | 182.97,78.11 182.96,78.42 JP9.1 JP6.2 173.36,78.42 7805.GND 173.36,72.07 173.36,71.76 C7.1 | 182.87,45.08 182.86,45.08 | S1.2 134.66,17.11 134.3,20.32 134.62,20.32 | 134.62,20.32 146.05,20.32 | 146.05,20.32 157.16,20.32 | R8.1 163.24,14.57 | R8.1 163.2,12.7 163.2,12.06 169.86,12.06 172.09,14.6 177.48,14.6 Q4.3 | S2.2 146.09,18.45 146.05,20.32 | S3.2 157.2,17.11 157.16,20.32 | S1.2 134.66,16.87 134.62,20.32 | 134.62,20.32 126.68,20.32 | 153.04,65.4 153.36,65.4 | 153.36,65.4 160.34,65.4 160.34,56.2 | 160.34,56.2 160.33,56.2 | C3.2 126.68,42.86 126.68,20.32
  Bottom 0.406: 126.68,20.32 126.68,22.23 C1.2 118.75,22.23 | LCD1.16 90.81,106.05 90.81,107.32 70.49,107.32 | 160.34,56.2 160.34,56.19 160.34,46.67 164.47,46.67 164.47,39.37 BUZZER.- | 157.16,20.32 157.17,19.37 163.2,19.37 163.2,14.57 163.16,14.57 R8.1 | 28PINS.8 70.17,24.45 | 70.17,24.45 70.17,19.37 | 70.17,19.37 28PINS.19 | 28PINS.19 | 28PINS.19 70.17,19.37 | C11.1 54.61,31.12 50.48,31.12 50.48,12.07 C9.1 | C9.1 55.25,0.47 50.17,0.47 49.85,0.48 | PICKIT_28.3 71.44,24.45 | 71.44,24.45 | 71.44,24.45 70.17,24.45 | 70.17,24.45 | LED7.K 164.79,107.32 165.1,107.64 165.1,111.49 165.42,111.49 | R9.1 59.37,57.79 59.37,58.42 v62.23,58.42 | C9.1 | 25.4,77.47 25.4,75.57 | 25.4,75.57 JP14.1 20.32,75.57 18.1,75.57 18.1,82.87 12.7,82.87 12.7,88.9 | LDR.2 22.86,107.32 v22.54,107.32 36.51,107.32 36.51,98.43 Q5.3 | v13.97,107.32 13.97,111.31 | C14.2 25.4,75.57 | 13.97,111.31 0.32,111.31 0.32,88.9 | 0.32,88.9 0.32,67.95 | 0.32,67.95 0.32,43.5 | 0.32,43.5 0.32,15.56 | 0.32,15.56 0.32,0.32 13.02,0.32 | R9.1 | R9.1 50.48,57.79 | 50.48,57.79 49.85,57.79 | 49.85,57.79 49.85,61.28 7.62,61.28 7.3,61.6 7.3,67.95 R25.1 | POTAR.1 20,94.02 20,88.9 12.7,88.9 | 12.7,88.9 0.32,88.9 | 27.94,0.32 28.26,0.32 | 33.02,0.32 13.02,0.32 | R25.1 R24.1 | R24.1 | R24.1 0.32,67.95 | R27.1 | R27.1 R26.1 v62.23,58.42 | R29.1 141.61,3.18 R28.1 141.61,0.32 129.54,0.32 | 33.02,25.4 | 33.02,25.4 33.02,30.48 37.46,30.48 40PINS.31 | 0.32,15.56 C12.1 4.44,15.56 4.44,20 C4.1 | C2.1 13.02,0.32 | S5.4 4.09,27.9 6.35,30.16 6.35,36.2 v4.76,37.78 | 0.32,43.5 0.63,43.18 v4.76,43.18 PICKIT_40.3 | 22.22,25.4 23.5,25.4 | 50.48,57.79 | C18.1 49.85,38.42 49.85,57.79 | S4.4 62.23,48.86 v62.23,48.9 | v62.23,58.42
  Bottom 0.406: C19.1 93.03,0.6 | 18PINS.5 103.51,26.67 103.51,7.62 114.94,7.62 PICKIT_18.3 114.93,5.08 114.93,0.39 | S6.4 88.58,9.6 v88.58,13.65 | v88.58,20.32 88.58,26.67 18PINS.5 | 18PINS.5 | C16.1 118.75,22.23 | 118.75,22.23 | 126.68,20.32 | R25.1 | C17.1 23.49,25.4 23.5,25.4 | LED3.K LED1.K LED2.K LED4.K LED5.K 153.04,65.08 153.36,65.4 | JP18.2 JP18.1 182.86,45.09 182.86,45.08 | MASSES.5 164.15,3.81 164.15,8.26 133.04,8.26 133.04,14.61 134.66,14.61 S1.2 | 70.17,19.37 | 70.17,19.37 70.17,4.45 C13.1 76.84,0.54
LED_POUSS
  Bottom 1.27: R12.1 JP2.2
N$1
  Bottom 1.27: 18PINS.16 113.67,31.75 113.67,36.51 121.16,36.51 | C3.1 121.16,36.51 | 121.16,36.51 Q3.2
N$2
  Bottom 1.27: 18PINS.11 JP3.3
N$3
  Bottom 1.27: 18PINS.15 116.53,29.21 | 116.53,29.21 119.07,29.21 | 119.07,29.21 | 119.07,29.21 122.24,29.21 C1.1 | Q3.1 116.53,31.75 116.53,29.21
N$4
  Bottom 1.27: 18PINS.10 JP3.4
N$5
  Bottom 1.27: JP3.1 18PINS.13 105.41,24.13 | 105.41,24.13 | 105.41,24.13 105.41,9.53 117.48,9.53 PICKIT_18.4 117.48,3.81 117.48,2.54 127.32,2.54 JP17.3
N$6  (via drill 0.6 pad 2.18)
  other vias: 10.8,20
N$7
  Bottom 1.27: PORTB1.1 18PINS.9
N$8  (via drill 0.6 pad 2.18)
  other vias: 7.3,13.02
N$9
  Bottom 1.27: PORTB1.3 18PINS.7
N$10
  Bottom 1.27: PORTB1.4 18PINS.6
N$11
  Bottom 1.27: PORT_A.5 111.44,43.18 111.44,34.29 18PINS.17
N$12
  Bottom 1.27: PORT_A.4 108.9,36.83 | 108.9,36.83 | 108.9,36.83 18PINS.18
N$13
  Bottom 0.406: 100.65,36.83 18PINS.1
  Bottom 1.27: 100.65,36.83 | PORT_A.3 | 100.65,36.83 104.14,36.83 106.37,39.05 PORT_A.3
N$14
  Bottom 1.27: 18PINS.2 98.11,34.29 98.11,39.69 103.19,39.69 103.83,40.32 PORT_A.2
N$15
  Bottom 1.27: 18PINS.3 95.57,31.75 95.57,42.86 99.7,42.86 PORT_A.1
N$16
  Bottom 1.27: PORT_B.1 40PINS.40 39.37,56.51 11.43,56.51 11.43,45.72 PICKIT_40.4 2.86,45.72 | JP15.1 2.86,45.72 | 2.86,45.72
N$17
  Bottom 1.27: 85.41,16.83 85.41,29.21 18PINS.4 | 85.41,16.83 85.41,9.6 S6.2 | C19.2 93.03,10.16 | 93.03,10.16 | 93.03,10.16 95.25,10.16 | 95.25,10.16 R1.1 | R1.1 95.25,10.16 | 95.25,10.16 93.03,10.16 | 93.03,10.16 93.03,16.83 85.41,16.83 | R1.1 100.65,10.16 100.65,5.08 PICKIT_18.1
N$18
  Bottom 1.27: PORT_B.2 40PINS.39 43.5,50.8 48.26,50.8 48.26,59.06 8.25,59.06 8.25,54.61 JP15.3 | JP15.3 5.4,48.26 | 5.4,48.26 | 5.4,48.26 PICKIT_40.5 | JP15.3
N$19
  Bottom 1.27: PICKIT_40.1 11.75,38.1 | 11.75,38.1 14.29,38.1 14.29,53.34 PORT_EA.10 40PINS.1 | R23.1 11.75,35.56 11.75,38.1 | R23.1 | S5.2 8.61,27.34 11.75,30.48 | 11.75,30.48 C17.2 | C17.2 | R23.1 11.75,30.48
N$20
  Bottom 1.27: LED1.A R12.2
N$21
  Bottom 1.27: S2.4 140.34,17.39 R4.1
N$22
  Bottom 1.27: 174.94,27.94 174.94,28.26 | 174.94,28.26 Q4.2 | 174.94,28.26 174.94,30.16 174.95,29.85 174.95,32.7 158.75,32.7 155.26,32.7 JP2.11
N$23
  Bottom 1.27: S3.4 151.45,17.39 R5.1
N$24
  Bottom 1.27: LED2.A R3.2
N$25
  Bottom 1.27: LED4.A R2.2
N$26
  Bottom 1.27: LED5.A R6.2
N$27
  Bottom 1.27: S1.4 128.91,17.39 R10.1
N$28  (via drill 0.6 pad 2.18)
  other vias: 133.99,2.86
N$29
  Bottom 1.27: S2.3 141.61,23.89 141.61,25.08 144.78,28.26 JP2.7
N$30  (1 unrouted)
  Bottom 1.27: JP2.8 147.32,28.26 151.77,23.81 152.6,23.81 S3.3 152.72,23.93
N$31
  Bottom 1.27: R8.2 | R8.2 163.51,22.22 R7.2 | 163.19,22.54 R8.2 | JP2.10 152.4,30.48 155.58,27.31 163.2,27.31 R8.2
N$32
  Bottom 1.27: R7.1 166.69,17.78 Q4.1
N$33
  Bottom 1.27: PORT_EA.9 40PINS.2
N$34
  Bottom 1.27: PORT_EA.8 40PINS.3
N$35
  Bottom 1.27: PORT_EA.7 40PINS.4 22.86,45.72
N$36
  Bottom 1.27: PORT_EA.6 40PINS.5
N$37
  Bottom 1.27: PORT_EA.5 40PINS.6
N$38
  Bottom 1.27: PORT_EA.4 40PINS.7
N$39
  Bottom 1.27: PORT_EA.3 40PINS.8
N$40
  Bottom 1.27: PORT_EA.2 40PINS.9
N$41
  Bottom 1.27: PORT_EA.1 40PINS.10
N$42
  Bottom 1.27: JP2.9 149.86,36.51 149.86,37.15 158.44,37.15 BUZZER.+
N$43  (via drill 0.6 pad 2.18)
  other vias: 12.38,13.02
N$44  (via drill 0.6 pad 2.18)
  other vias: 13.02,7.94
N$45  (via drill 0.6 pad 2.18)
  other vias: 97.48,10.16
N$46  (via drill 0.6 pad 2.18)
  other vias: 97.48,2.54
N$47  (via drill 0.6 pad 2.18)
  other vias: 122.24,27.31
N$48  (via drill 0.6 pad 2.18)
  other vias: 116.21,32.39
N$49  (via drill 0.6 pad 2.18)
  other vias: 121.29,32.39
N$50  (via drill 0.6 pad 2.18)
  other vias: 121.29,37.78
N$51  (via drill 0.6 pad 2.18)
  other vias: 93.03,8.89
N$52  (via drill 0.6 pad 2.18)
  other vias: 133.99,5.4
N$53  (via drill 0.6 pad 2.18)
  other vias: 140.34,13.02
N$54  (via drill 0.6 pad 2.18)
  other vias: 147.96,13.02
N$55  (via drill 0.6 pad 2.18)
  other vias: 128.91,13.02
N$56  (via drill 0.6 pad 2.18)
  other vias: 159.07,13.02
N$57  (via drill 0.6 pad 2.18)
  other vias: 163.2,22.23
N$58  (via drill 0.6 pad 2.18)
  other vias: 166.69,22.23
N$59  (via drill 0.6 pad 2.18)
  other vias: 166.69,14.61
N$60  (via drill 0.6 pad 2.18)
  other vias: 132.08,55.25
N$61  (via drill 0.6 pad 2.18)
  other vias: 139.07,55.25
N$62  (via drill 0.6 pad 2.18)
  other vias: 146.05,55.25
N$63  (via drill 0.6 pad 2.18)
  other vias: 153.04,55.25
N$64  (via drill 0.6 pad 2.18)
  other vias: 136.53,13.02
N$65  (via drill 0.6 pad 2.18)
  other vias: 118.75,25.08
N$66  (via drill 0.6 pad 2.18)
  other vias: 40.64,104.46
N$67  (via drill 0.6 pad 2.18)
  other vias: 153.04,47.63
N$68
  Bottom 1.27: 40PINS.38 PORT_B.3
N$69
  Bottom 1.27: 40PINS.37 PORT_B.4
N$70
  Bottom 1.27: 40PINS.36 PORT_B.5
N$71
  Bottom 1.27: 40PINS.35 PORT_B.6
N$72
  Bottom 1.27: 40PINS.34 PORT_B.7
N$73
  Bottom 1.27: 40PINS.33 PORT_B.8
N$74
  Bottom 1.27: JP11.6 17.14,17.78 40PINS.15
N$75
  Bottom 1.27: JP11.5 18.73,13.34 20.64,15.24 40PINS.16
N$76
  Bottom 1.27: JP11.4 19.37,10.8 21.27,12.7 40PINS.17
N$77
  Bottom 1.27: JP11.2 20.96,5.72 22.86,7.62 40PINS.19
N$78
  Bottom 1.27: JP11.1 23.81,3.18 24.13,3.49 40PINS.20
N$79
  Bottom 1.27: 40PINS.30 PORT_CD2.1
N$80
  Bottom 1.27: 40PINS.29 PORT_CD2.2
N$81
  Bottom 1.27: 40PINS.27 PORT_CD2.4
N$82
  Bottom 1.27: 40PINS.28 PORT_CD2.3
N$83
  Bottom 1.27: PORT_CD2.5 40PINS.26
N$84
  Bottom 1.27: 40PINS.25 PORT_CD2.6
N$85
  Bottom 1.27: PORT_CD2.7 40PINS.24
N$86
  Bottom 1.27: 40PINS.23 PORT_CD2.8
N$87
  Bottom 1.27: PORT_CD2.9 40PINS.22
N$88
  Bottom 1.27: 40PINS.21 PORT_CD2.10
N$89
  Bottom 1.27: LCD1.3 57.79,97.48 55.25,97.48 55.25,60.64 54.61,60.64 R9.2
N$90
  Bottom 1.27: 40PINS.14 14.92,20.32 12.38,17.34 Q1.2 13.02,13.02 13.02,11.75 C2.2
N$91
  Bottom 1.27: 40PINS.13 13.65,22.86 C4.2 | Q1.1 7.43,16.95 C4.2 | C4.2
N$92  (via drill 0.6 pad 2.18)
  other vias: 146.05,47.63
N$93
  Bottom 1.27: 8X8_A2.7 8X8_A1.2
N$94
  Bottom 1.27: 8X8_A1.3 8X8_A2.6
N$95
  Bottom 1.27: 8X8_A1.4 8X8_A2.5
N$96
  Bottom 1.27: 8X8_A2.4 8X8_A1.5
N$97
  Bottom 1.27: 8X8_A1.6 8X8_A2.3
N$98
  Bottom 1.27: 8X8_A2.2 8X8_A1.7
N$99
  Bottom 1.27: 8X8_A1.8 8X8_A2.1
N$100
  Bottom 1.27: 8X8_B2.1 8X8_B1.8
N$101
  Bottom 1.27: 8X8_B1.7 8X8_B2.2
N$102
  Bottom 1.27: 8X8_B2.3 8X8_B1.6
N$103
  Bottom 1.27: 8X8_B1.5 8X8_B2.4
N$104
  Bottom 1.27: 8X8_B2.5 8X8_B1.4
N$105
  Bottom 1.27: 8X8_B1.3 8X8_B2.6
N$106
  Bottom 1.27: 8X8_B2.7 8X8_B1.2
N$107
  Bottom 1.27: 8X8_B1.1 8X8_B2.8
N$108
  Bottom 1.27: LCD1.11 78.11,99.7 67.95,99.7 LCD.4
N$109
  Bottom 1.27: LCD1.4 | LCD1.4 LCD.7
N$110
  Bottom 1.27: LCD1.5 | LCD1.5 LCD.6
N$111
  Bottom 1.27: 65.41,67.94 LCD.5 65.41,67.94 LCD1.6
N$112
  Bottom 1.27: LCD.3 70.49,67.94 70.49,96.84 80.65,96.84 LCD1.12
N$113
  Bottom 1.27: LCD.2 73.03,67.94 73.03,93.98 83.19,93.98 LCD1.13
N$114
  Bottom 1.27: LCD.1 75.57,67.94 75.57,91.13 85.73,91.13 LCD1.14
N$115  (via drill 0.6 pad 2.18)
  other vias: 151.45,13.02
N$116
  Bottom 1.27: JP2.5 139.7,36.2 139.7,40.01 153.04,40.01 153.04,47.3 R6.1
N$117
  Bottom 1.27: 130.18,23.89 S1.3 130.18,23.93 130.18,26.67 139.39,26.67 142.24,29.53 JP2.6
N$118
  Bottom 1.27: R2.1 | R2.1 | R2.1 | R2.1 | JP2.4 137.16,42.55 146.05,42.55 R2.1
N$119
  Bottom 1.27: R3.1 139.07,45.4 134.62,45.4 JP2.3
N$120  (via drill 0.6 pad 2.18)
  other vias: 139.07,47.63
N$121  (via drill 0.6 pad 2.18)
  other vias: 132.08,47.63
N$122  (via drill 0.6 pad 2.18)
  other vias: 132.08,60.01
N$123  (via drill 0.6 pad 2.18)
  other vias: 139.07,60.01
N$124  (via drill 0.6 pad 2.18)
  other vias: 146.05,60.01
N$125  (via drill 0.6 pad 2.18)
  other vias: 153.04,60.01
N$126  (via drill 0.6 pad 2.18)
  other vias: 158.44,39.37
N$127  (via drill 0.6 pad 2.18)
  other vias: 167.01,64.14
N$128  (via drill 0.6 pad 2.18)
  other vias: 169.23,71.76
N$129  (via drill 0.6 pad 2.18)
  other vias: 171.46,75.88
N$130  (via drill 0.6 pad 2.18)
  other vias: 171.46,78.74
N$131  (via drill 0.6 pad 2.18)
  other vias: 174,89.22
N$132  (via drill 0.6 pad 2.18)
  other vias: 174,86.36
N$133  (via drill 0.6 pad 2.18)
  other vias: 171.46,92.71
N$134  (via drill 0.6 pad 2.18)
  other vias: 171.46,82.55
N$135  (via drill 0.6 pad 2.18)
  other vias: 160.66,107.32
N$136  (via drill 0.6 pad 2.18)
  other vias: 148.91,107.32
N$137  (via drill 0.6 pad 2.18)
  other vias: 66.36,109.54
N$138  (via drill 0.6 pad 2.18)
  other vias: 78.42,109.54
N$139  (via drill 0.6 pad 2.18)
  other vias: 157.8,71.12
N$140  (via drill 0.6 pad 2.18)
  other vias: 157.8,61.91
N$141  (via drill 0.6 pad 2.18)
  other vias: 167.33,48.58
N$142
  Top 0.1: 102.56,49.85 105.41,49.85
N$143
  Bottom 1.27: R13.2 LED7.A | LED7.A
N$144
  Bottom 1.27: LCD1.15 88.27,103.82 88.27,100.02 131.45,100.02 R14.1
N$145
  Bottom 1.27: R14.2 3.3V1.2 | 3.3V1.2
N$146  (via drill 0.6 pad 2.18)
  other vias: 156.53,107.32
N$147  (via drill 0.6 pad 2.18)
  other vias: 131.45,104.78
N$148  (1 unrouted)
  Bottom 1.27: JP7.1 91.44,65.09 JP7.1 | JP8.7 94.3,65.09
N$149  (1 unrouted)
  Bottom 1.27: JP8.6 94.3,62.55 | JP7.2 91.44,62.55
N$150  (1 unrouted)
  Bottom 1.27: JP7.3 91.44,60.01 | JP8.5 94.3,60.01
N$151  (1 unrouted)
  Bottom 1.27: JP7.4 91.44,57.47 | JP8.4 94.62,57.47
N$152  (1 unrouted)
  Bottom 1.27: JP7.5 91.12,54.93 | JP8.3 94.62,54.93
N$153  (1 unrouted)
  Bottom 1.27: JP10.7 110.17,65.09 110.18,65.09 | JP5.1 113.35,65.09
N$154  (1 unrouted)
  Bottom 1.27: JP10.6 110.49,62.55 | JP5.2 113.35,62.55
N$155  (1 unrouted)
  Bottom 1.27: JP5.3 113.35,60.01 | JP10.5 110.81,60.01
N$156  (1 unrouted)
  Bottom 1.27: JP10.4 110.81,57.47 | JP5.4 113.35,57.47
N$157  (1 unrouted)
  Bottom 1.27: JP10.3 110.81,54.93 | JP5.5 113.35,54.93
N$158  (1 unrouted)
  Bottom 1.27: JP7.6 91.12,52.39 | JP8.2 94.62,52.39
N$159  (1 unrouted)
  Bottom 1.27: JP7.7 91.12,49.85 | JP8.1 94.3,49.85
N$160  (1 unrouted)
  Bottom 1.27: JP5.6 113.35,52.39 | JP10.2 110.81,52.39
N$161  (1 unrouted)
  Bottom 1.27: JP10.1 110.81,49.85 | JP5.7 113.35,49.85
N$162  (via drill 0.6 pad 2.18)
  other vias: 139.07,104.78
N$163  (via drill 0.6 pad 2.18)
  other vias: 52.07,62.87
N$164  (via drill 0.6 pad 2.18)
  other vias: 125.1,47.63
N$165  (via drill 0.6 pad 2.18)
  other vias: 33.02,104.46
N$166
  Bottom 1.27: C9.2 55.25,21.91 Q2.2 56.83,21.91 59.37,19.37 28PINS.10
N$167
  Bottom 1.27: 60.64,21.91 28PINS.9 | 28PINS.9 | Q2.1 60.64,21.91 | 60.64,21.91 55.88,26.35 | 55.88,26.35 | 55.88,26.35 C11.2
N$168
  Bottom 1.27: RA.6 28PINS.2
N$169  (via drill 0.6 pad 2.18)
  other vias: 58.74,45.72
N$170
  Bottom 1.27: RA.5 28PINS.3
N$171
  Bottom 0.406: 28PINS.28
  Bottom 1.27: PICKIT_28.4 28PINS.28 | 28PINS.28 | 28PINS.28 RB.1 | JP16.1 79.69,53.02 | 79.69,53.02 | 79.69,53.02 73.98,53.02 PICKIT_28.4 | PICKIT_28.4
N$172  (1 unrouted)
  Bottom 0.406: 78.42,39.05 78.42,39.37
  Bottom 1.27: 28PINS.27 RB.2 | RB.2 | PICKIT_28.5 76.52,49.21 76.52,45.72 82.55,45.72 | 82.55,45.72 82.55,39.69 RB.2 | RB.2 | 82.55,45.72 82.55,60.96 JP16.3 | JP16.3
N$173
  Bottom 1.27: RA.4 28PINS.4
N$174
  Bottom 1.27: RA.3 28PINS.5
N$175
  Bottom 1.27: RA.2 28PINS.6
N$176
  Bottom 1.27: RA.1 28PINS.7
N$177
  Bottom 1.27: RC.4 59.69,16.83 | 59.69,16.83 | 59.69,16.83 28PINS.11
N$178
  Bottom 1.27: RC.3 61.28,12.7 62.87,14.29 28PINS.12
N$179
  Bottom 1.27: RC.2 62.23,10.16 63.82,11.75 28PINS.13
N$180
  Bottom 1.27: RC.1 63.5,7.62 65.09,9.21 28PINS.14
N$181
  Bottom 1.27: 28PINS.18 79.06,16.83 RC2.1
N$182
  Bottom 1.27: 28PINS.17 79.06,14.29 RC2.2
N$183
  Bottom 1.27: 28PINS.16 79.06,11.75 RC2.3
N$184
  Bottom 1.27: 28PINS.15 79.06,9.21 RC2.4
N$185
  Bottom 1.27: 28PINS.21 RB.8 | RB.8
N$186
  Bottom 1.27: 28PINS.22 RB.7 | RB.7
N$187
  Bottom 1.27: 28PINS.23 RB.6 | RB.6
N$188
  Bottom 1.27: 28PINS.24 RB.5 | RB.5
N$189
  Bottom 1.27: 28PINS.25 RB.4 | RB.4
N$190
  Bottom 1.27: 28PINS.26 RB.3 | RB.3
N$191  (via drill 0.6 pad 2.18)
  other vias: 54.61,60.33
N$192  (via drill 0.6 pad 2.18)
  other vias: 55.25,26.35
N$193  (via drill 0.6 pad 2.18)
  other vias: 55.25,21.91
N$194  (via drill 0.6 pad 2.18)
  other vias: 60.33,21.91
N$195  (via drill 0.6 pad 2.18)
  other vias: 55.25,17.15
N$196
  Bottom 1.27: POTAR.2 30.48,96.52 30.48,78.11 33.34,78.11 JP4.5
N$197  (via drill 0.6 pad 2.18)
  Bottom 1.27: 21.27,66.99 R17.2 | R17.2 | R17.2 | 21.27,66.99 C14.1 27.94,66.99 27.94,73.03 33.34,73.03 JP4.3 | 21.27,66.99
  Bottom 3.81: JP13.1 21.27,69.85 | 21.27,69.85 21.27,71.12 | 21.27,69.85 21.27,66.99
  other vias: 17.46,66.99
N$198  (via drill 0.6 pad 2.18)
  Bottom 1.27: R18.2 | R18.2 21.27,85.09 | JP12.1 21.27,85.73 20.96,85.73 20.96,85.41 C15.1 27.94,85.41 27.94,75.57 JP4.4 | JP4.4
  Bottom 3.81: JP12.1 | JP12.1 21.27,80.01 | JP12.1 21.27,85.09
  other vias: 17.46,85.09
N$199
  Bottom 1.27: LDR.1 R16.2 33.66,104.46 JP4.6
N$200  (via drill 0.6 pad 2.18)
  other vias: 19.69,96.52
N$201  (via drill 0.6 pad 2.18)
  other vias: 37.15,95.57
N$202  (via drill 0.6 pad 2.18)
  other vias: 39.37,97.16
N$203  (via drill 0.6 pad 2.18)
  other vias: 30.48,104.46
N$204  (via drill 0.6 pad 2.18)
  other vias: 25.4,66.99
N$205  (via drill 0.6 pad 2.18)
  other vias: 25.4,85.41
N$206  (via drill 0.6 pad 2.18)
  Bottom 1.27: LED3.A | LED3.A R19.2 | R19.2 125.1,57.79 R19.2
  other vias: 125.1,55.25 125.1,60.01
N$207
  Bottom 1.27: R19.1 125.1,46.04 125.1,45.09 129.54,45.09 129.54,36.51 JP2.1
N$208  (via drill 0.6 pad 2.18)
  Bottom 1.27: Q5.2 42.23,97.16 R21.2 | R21.2 | R21.2 42.23,67.95 JP4.1 | JP4.1
  other vias: 42.23,92.4
N$209  (via drill 0.6 pad 2.18)
  Bottom 1.27: Q5.1 | Q5.1 R20.2 | R20.2
  other vias: 37.15,91.76
N$210
  Bottom 1.27: JP4.2 37.15,70.49 R20.1
N$211
  Bottom 1.27: JP11.3 20.32,8.26 22.23,10.16 40PINS.18
N$212  (via drill 0.6 pad 2.18)
  other vias: 66.36,45.72
N$213
  Bottom 1.27: PICKIT_28.1 66.36,46.99 | 28PINS.1 | 28PINS.1 66.36,46.99 | 66.36,46.99 R22.1 | S4.2 66.32,53.38 66.36,53.34 PICKIT_28.1 | PICKIT_28.1 | C18.2 55.56,42.23 | 55.56,42.23 | 55.56,42.23 28PINS.1
N$214  (via drill 0.6 pad 2.18)
  other vias: 14.29,30.48
N$215  (via drill 0.6 pad 2.18)
  other vias: 11.75,40.64
N$216
  Bottom 1.27: R24.2 2.86,57.47 JP15.2
N$217
  Bottom 1.27: R25.2 5.4,57.47 JP15.4
N$218  (via drill 0.6 pad 2.18)
  other vias: 5.4,60.33
N$219  (via drill 0.6 pad 2.18)
  other vias: 2.86,60.33
N$220  (via drill 0.6 pad 2.18)
  other vias: 11.75,33.02
N$221  (via drill 0.6 pad 2.18)
  other vias: 37.15,84.14
N$222
  Bottom 1.27: JP16.2 72.39,58.42 R26.2
N$223  (via drill 0.6 pad 2.18)
  Bottom 1.27: R27.2 | R27.2 | R27.2 JP16.4
  other vias: 72.07,60.96
N$224
  Bottom 1.27: JP17.4 129.86,2.86 R28.2
N$225
  Bottom 1.27: JP17.2 129.86,5.4 R29.2
N$226  (via drill 0.6 pad 2.18)
  other vias: 72.07,58.42
N$227  (via drill 0.6 pad 2.18)
  other vias: 1.9,20.64
PORT_B84
  Bottom 1.27: PORTB1.2 18PINS.8
PORTB2
  Bottom 1.27: 18PINS.12 JP3.2 116.84,21.59 116.84,12.07 | 116.84,12.07 120.02,12.07 PICKIT_18.5 | JP17.1 126.05,5.4 126.05,12.07 116.84,12.07
V+  (via drill 0.6, 0.6 pad 2.18)
  Top 1.27: v66.36,109.54 v78.42,109.54 | v157.8,71.12 v157.8,61.91
  Bottom 1.27: 7805XL.OUT 167.32,53.66 C5.2 167.32,45.09 167.33,45.09 171.14,45.09 | v66.36,109.54 55.25,109.54 LCD1.2 55.25,100.02 52.39,100.02 | 145.1,107.32 JP1.5 JP1.4 JP1.3 JP1.2 JP1.1 133.04,109.22 133.04,109.54 78.11,109.54 v78.42,109.54 | 145.1,107.32 3.3V1.1 145.1,71.44 145.1,71.12 151.76,71.12 v157.8,71.12 | 170.5,36.2 170.5,45.09 170.5,45.08 171.14,45.08 171.14,45.09 | 170.5,36.2 167.64,36.2 | 145.1,107.32 148.28,107.32 | 148.28,107.32 | 148.28,107.32 R13.1 | R13.1 | R17.1 | 42.23,104.46 42.23,109.86 19.69,109.86 v19.69,99.06 19.69,99.02 POTAR.3 | R21.1 52.39,100.02 | R18.1 | R18.1 3.17,85.09 3.17,70.17 9.84,70.17 R17.1 | R17.1 10.16,66.99 | R17.1 | 52.07,63.5 9.84,63.5 R17.1 | R16.1 42.23,104.46 | 42.23,104.46 R21.1 | 170.5,36.2 167.32,36.2 162.25,36.2 162.25,43.18 157.8,43.18 v157.8,61.91 | R21.1 | 52.07,63.5 R9.3 | 52.07,63.5 52.39,63.5 52.39,100.02 | 171.14,45.09 JP18.3 | JP18.3 | JP18.3 174.31,40.64 180.66,40.64 180.66,12.07 174.31,12.07 170.82,10.16 159.07,10.16 | R10.2 136.53,10.16 | 136.53,10.48 136.53,10.16 | 136.53,10.16 147.96,10.16 | 147.96,10.16 | 147.96,10.16 R4.2 147.96,10.16 | 147.96,10.47 147.96,10.16 | 147.96,10.16 159.07,10.16 | 159.07,10.16 R5.2 | 159.07,10.16
  other vias: 9.84,85.09 9.84,66.99 42.23,100.02
VCC/2
  Bottom 1.27: 7803.OUT 171.45,88.9 C10.2 171.45,95.57 178.44,95.57 3.3V.1

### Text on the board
Bottom: Platine école PIC V.3 / F6FCO
tTest: Vcc disponibles | a0 | a1 | a2 | a3 | a4 | a0 | a4 | a3 | a2 | a1 | a0 | a5 | a1 | a2 | a3 | a4 | a5
Holes: e0 | e1 | e2 | Gnd disponibles
Milling: c7 | c7 | c0 | c6 | c0 | c6 | c1 | c5 | c1 | c2 | c5 | c4 | c2 | c4 | c3 | c3
Document: Sortie 3.3v | LCD | Matrice Led / 8x8 | Platine école PIC V.2 / - F6FCO - | Ldr | Pot | Enc1 | Entrée / alim 6/12vcc | Enc2 | NPN_e | Rs | R/W | E | D4 | D5 | D6 | D7 | Afficheur / 7 seg | NPN_s | Led1 | Led2 | Led3 | Led4 | Led5 | b7 | Mclr | Vdd | Gnd | Pgd | Pgc | b6 | Pgc | b5 | Raz | Pgd | b4 | Sortie 5vcc | Gnd | b3 | b7 | Vdd | b2 | b6 | Mclr | Pickit 40pins | b1 | b5 | b0 | b4 | Led1 | Led2 | Led3 | Led4 | Led5 | P1 | P2 | P3 | Buzzer | TTor g | TTor d | b3 | b2 | b1 | Raz | b0 | b0 | b7 | P1 | P2 | P3 | P4 | b1 | b6 | b2 | b5 | b3 | b4 | Pickit 18pins | Raz | Mclr | Vdd | Gnd | Pgd | Pgc
Reference: 1 | 16 | 8 | 9 | k | d7 | d6 | d5 | d4 | d3 | d0 | d2 | d1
